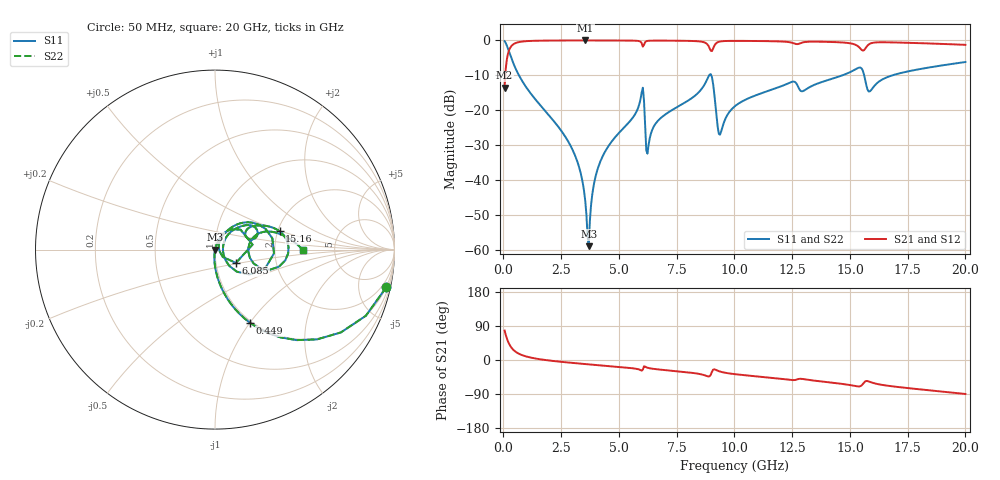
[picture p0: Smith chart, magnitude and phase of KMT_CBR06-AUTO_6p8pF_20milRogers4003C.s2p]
! Data measured by Modelithics Inc. support@modelithics.com 813-866-6335
! KEMET CBR06-AUTO 6.8pF, Pad Width= 0.851mm, Pad Length= 0.64mm, Pad Gap= 0.62mm, 20mil Rogers 4003C substrate Data, January 2022
# hz S ma R 50
! 2 Port Network Data from SP1.SP block
! freq  magS11  angS11  magS21  angS21  magS12  angS12  magS22  angS22
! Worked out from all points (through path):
!   401 points, 50 MHz to 20 GHz, reference 50 ohm
!   highest |S21| = -0.01 dB at 3.541 GHz (marker M1); lowest = -13.5 dB at 50 MHz (marker M2)
!   group delay of S21, straight-line fit = 13.9 ps
!   lowest |S11| = -58.8 dB at 3.691 GHz (marker M3), VSWR 1.00, Z = 50.1 + j0.0373 ohm
!   |S11| at or under -10 dB: 673.6 MHz to 8.906 GHz (8.232 GHz wide, 172 % of centre); 8.999 GHz to 14.66 GHz (5.664 GHz wide, 47.9 % of centre); 15.62 GHz to 16.83 GHz (1.209 GHz wide, 7.45 % of centre)
!   |S22| runs from -58.8 to -0.2 dB; largest |S21 - S12| = 0
!   S11 on the Smith chart (normalised r, x): 50 MHz: 0.98, -9.16; 449 MHz: 0.98, -1.01; 6.085 GHz: 1.25, -0.19; 15.16 GHz: 2.05, +0.48; 20 GHz: 2.93, -0.02
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5e7  0.9775 -12.3  0.2108 77.7  0.2108 77.7  0.9775 -12.3
2.495e8  0.6789 -48.0  0.7337 42.0  0.7337 42.0  0.6789 -48.0
4.49e8  0.4535 -64.4  0.8907 25.6  0.8907 25.6  0.4535 -64.4
2.74325e9  0.03885 -95.0  0.9983 -6.3  0.9983 -6.3  0.03885 -95.0
3.391625e9  0.01082 -94.9  0.9989 -9.9  0.9989 -9.9  0.01082 -94.9
3.54125e9  0.005107 -89.8  0.9989 -10.7  0.9989 -10.7  0.005107 -89.8
3.690875e9  0.001149 18.9  0.9989 -11.5  0.9989 -11.5  0.001149 18.9
3.94025e9  0.009671 71.1  0.9988 -12.8  0.9988 -12.8  0.009671 71.1
4.289375e9  0.02194 72.5  0.9985 -14.6  0.9985 -14.6  0.02194 72.5
5.985125e9  0.1807 38.0  0.9126 -28.0  0.9126 -28.0  0.1807 38.0
6.084875e9  0.1383 -32.4  0.866 -16.7  0.866 -16.7  0.1383 -32.4
6.284375e9  0.0322 48.9  0.9884 -21.2  0.9884 -21.2  0.0322 48.9
6.73325e9  0.0737 62.6  0.994 -25.0  0.994 -25.0  0.0737 62.6
8.92775e9  0.3256 11.2  0.7727 -42.8  0.7727 -42.8  0.3256 11.2
9.376625e9  0.04499 8.8  0.9645 -30.5  0.9645 -30.5  0.04499 8.8
1.0025e10  0.1151 48.8  0.9854 -37.4  0.9854 -37.4  0.1151 48.8
1.336662e10  0.2247 32.7  0.9602 -53.8  0.9602 -53.8  0.2247 32.7
1.516212e10  0.3742 15.7  0.8866 -68.0  0.8866 -68.0  0.3742 15.7
1.551125e10  0.3956 -8.9  0.7309 -66.7  0.7309 -66.7  0.3956 -8.9
1.586038e10  0.1869 3.3  0.895 -57.6  0.895 -57.6  0.1869 3.3
1.670825e10  0.3067 19.2  0.939 -68.5  0.939 -68.5  0.3067 19.2
2e10  0.4913 -0.3  0.8646 -89.7  0.8646 -89.7  0.4913 -0.3
